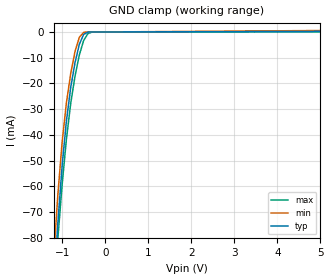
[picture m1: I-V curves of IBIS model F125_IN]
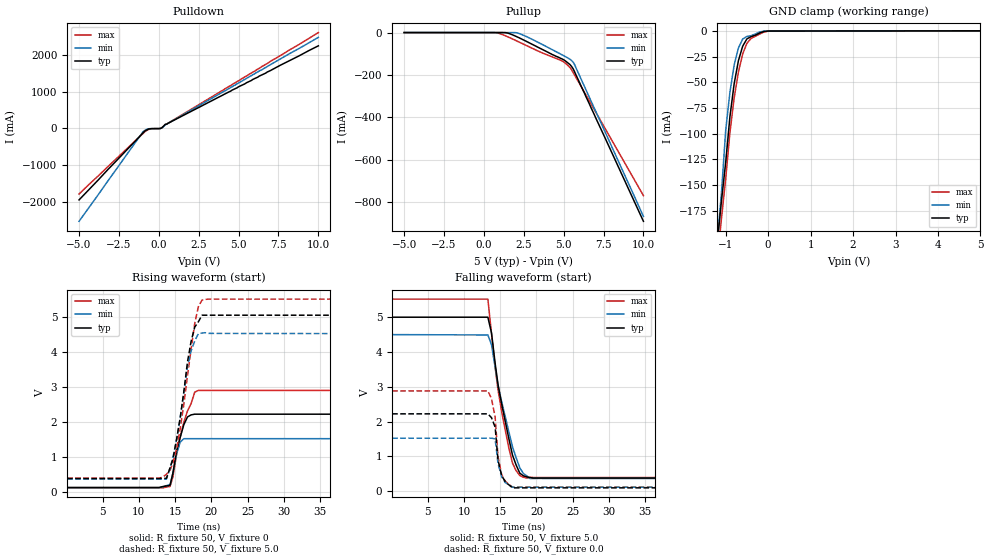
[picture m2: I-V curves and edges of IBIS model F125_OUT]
| TEXAS INSTRUMENTS INCORPORATED
| Standard Linear and Logic Group
| IBIS Model of SN74F125
| QUADRUPLE BUS BUFFER GATE WITH 3-STATE OUTPUTS
| SOIC 14-pin (D),PDIP 14-pin (N), SOP 14-pin (NS) Package.
[IBIS Ver]   3.2
[Comment Char]  |_char
[File Name]   sn74f125.ibs
[File Rev]   3.1
[Date]   Nov. 03, 2004
[Source]   Data created from Lab data at TI-SLL.
[Notes]   The following is an IBIS list for the F125.
   - FILE REV HISTORY
   - 3.1 Re-Release IBIS file on 11/03/04
   - Power clamp data deleted as there is no power-clamp diode.
|   Please contact sllibis@ti.com with questions and
|   comments concerning SLL IBIS models.
[Disclaimer] Property of Texas Instruments Incorporated.  Unauthorized
   reproduction and/or distribution is strictly prohibited.
   This product is protected under copyright law.
   Created 2000, (C) Copyright 2000, Texas Instruments Inc.,
   All Rights Reserved.
   UNLESS THERE IS A SIGNED, WRITTEN AGREEMENT TO THE
   CONTRARY, TEXAS INSTRUMENTS () IS PROVIDING THE IBIS
   MODELS  AND WITHOUT ANY WARRANTY, EXPRESSED OR
   IMPLIED.  TI assumes no liability for:
   1) the accuracy of the IBIS models provided to your
   company;
   2) the proper functioning of these IBIS Models in your
   design or for any resulting applications; or
   3) infringement of patents, copyrights or intellectual
   property rights resulting from your use of these IBIS
   models.
   TI provides IBIS Models as a service to our customers.
   You and your company shall not distribute, sell or give
   these models to anyone else without prior written
   permission from TI.
   TI reserves the right to make changes to our products or
   to discontinue any semiconductor product or service
   without notice, and advises our customers to obtain the
   latest version of relevant information to verify, before
   placing orders, that the information being relied on is
   current.
   Please be aware that your receipt and use of the IBIS
   information provided shall serve as acceptance of these
   terms and conditions.  If you do not accept these terms,
   you should return or destroy the IBIS models and any
   other accompanying information immediately.
|   Component F125_D
[Component]   F125_D
[Manufacturer]  Texas Instruments Incorporated
[Package]
|   Typ.   Min.   Max.
R_pkg   0.031   0.028   0.034
L_pkg   3.109nH   2.462nH   3.889nH
C_pkg   0.473pF   0.363pF   0.628pF
[Pin]   Signal_name   Model_name   R_pin   L_pin   C_pin
1   1OE_NOT   F125_IN   0.033   3.854nH   0.622pF
2   1A   F125_IN   0.032   3.188nH   0.473pF
3   1Y   F125_OUT   0.028   2.462nH   0.377pF
4   2OE_NOT   F125_IN   0.031   2.596nH   0.363pF
5   2A   F125_IN   0.028   2.521nH   0.372pF
6   2Y   F125_OUT   0.034   3.25nH   0.476pF
7   GND   GND   0.034   3.889nH   0.628pF
8   3Y   F125_OUT   0.034   3.889nH   0.628pF
9   3A   F125_IN   0.034   3.25nH   0.476pF
10   3OE_NOT   F125_IN   0.028   2.521nH   0.372pF
11   4Y   F125_OUT   0.031   2.596nH   0.364pF
12   4A   F125_IN   0.028   2.462nH   0.377pF
13   4OE_NOT   F125_IN   0.032   3.188nH   0.473pF
14   VCC   POWER   0.033   3.854nH   0.622pF
|   Component F125_N
[Component]   F125_N
[Manufacturer]  Texas Instruments Incorporated
[Package]
|   Typ.   Min.   Max.
R_pkg   0.045   0.037   0.063
L_pkg   5.407nH   3.922nH   6.942nH
C_pkg   0.389pF   0.205pF   0.604pF
[Pin]  Signal_name   Model_name   R_pin   L_pin   C_pin
1   1OE_NOT   F125_IN   0.063   6.942nH   0.604pF
2   1A   F125_IN   0.037   6.2nH   0.406pF
3   1Y   F125_OUT   0.042   4.389nH   0.322pF
4   2OE_NOT   F125_IN   0.038   3.922nH   0.205pF
5   2A   F125_IN   0.039   4.301nH   0.298pF
6   2Y   F125_OUT   0.038   5.329nH   0.356pF
7   GND   GND   0.053   6.51nH   0.544pF
8   3Y   F125_OUT   0.053   6.437nH   0.539pF
9   3A   F125_IN   0.039   5.352nH   0.347pF
10   3OE_NOT   F125_IN   0.042   4.473nH   0.297pF
11   4Y   F125_OUT   0.044   4.326nH   0.225pF
12   4A   F125_IN   0.042   4.295nH   0.28pF
13   4OE_NOT   F125_IN   0.042   6.318nH   0.418pF
14   VCC   POWER   0.061   6.9nH   0.603pF
|   Component F125_NS
[Component]   F125_NS
[Manufacturer]  Texas Instruments, Inc.
[Package]
|   typ   min   max
R_pkg   4.500e-02   3.900e-02   5.400e-02
L_pkg   3.796e-09   2.561e-09   4.952e-09
C_pkg   5.280e-13   2.880e-13   7.100e-13
[Pin]   signal_name   model_name   R_pin   L_pin   C_pin
1   1OE_NOT   F125_IN   4.700e-02   4.867e-09   7.060e-13
2   1A   F125_IN   5.100e-02   4.083e-09   5.920e-13
3   1Y   F125_OUT   4.100e-02   2.915e-09   3.760e-13
4   2OE_NOT   F125_IN   3.900e-02   2.561e-09   2.880e-13
5   2A   F125_IN   4.100e-02   3.101e-09   4.300e-13
6   2Y   F125_OUT   4.700e-02   4.047e-09   5.890e-13
7   GND   GND   5.100e-02   4.909e-09   7.000e-13
8   3Y   F125_OUT   4.500e-02   4.784e-09   6.940e-13
9   3A   F125_IN   5.400e-02   4.176e-09   5.970e-13
10   3OE_NOT   F125_IN   3.900e-02   3.287e-09   4.490e-13
11   4Y   F125_OUT   3.900e-02   2.586e-09   2.940e-13
12   4A   F125_IN   4.000e-02   2.802e-09   3.710e-13
13   4OE_NOT   F125_IN   4.900e-02   4.080e-09   5.930e-13
14   VCC   POWER   5.200e-02   4.952e-09   7.100e-13
| Models and submodels in the file (2): F125_IN (Input), F125_OUT (3-state)
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|   Model F125_IN
[Model]   F125_IN
Model_type  Input
Polarity   Inverting
Vinl = 0.8
Vinh = 2.0
| variable   typ   min   max
C_comp   1.24pf   0.94pf   1.54pf
[Temperature Range]   25   0   70
[Voltage Range]   5.0   4.5   5.5
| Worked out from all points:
|   GND clamp passes 1 mA (typ) near -0.50 V on its own axis
[GND Clamp]
|   Voltage   I(typ)   I(min)   I(max)
-5V       -1.74A     -1.55A     -1.51A
-1.2V     -101mA     -88.7mA    -104mA
-1.1V     -74.4mA    -63.5mA    -80.4mA
-1V       -52mA      -42.8mA    -59.4mA
-900mV    -34.5mA    -27.5mA    -41.6mA
-800mV    -21.5mA    -16.1mA    -27.7mA
-700mV    -11.9mA    -7.52mA    -17.1mA
-600mV    -4.79mA    -2.08mA    -8.9mA
-500mV    -950uA     -140uA     -3.31mA
-400mV    -55.2uA    -3.23uA    -617uA
-300mV    -1.95uA    -61.9nA    -49uA
5V        230uA      555uA      4.72uA
|   Model F125_OUT
[Model]   F125_OUT
Model_type  3-state
Polarity   Non-Inverting
Enable   Active-High
Vmeas = 2.5v
Cref = 15pf
| variable   typ   min   max
C_comp   6.5pf   4.87pf   8.13pf
[Temperature Range]   25   0   70
[Voltage Range]   5.0   4.5   5.5
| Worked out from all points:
|   slope of the pulldown table from 0 to 0.75 V, typ, clamps not added: 4.12 ohm
|   GND clamp passes 1 mA (typ) near -0.14 V on its own axis
|   rising waveform, R_fixture 50, V_fixture 0: 20-80 % time 1.33ns typ, 901ps min, 1.89ns max; typ from 0.125 V to 2.22 V
|   falling waveform, R_fixture 50, V_fixture 5.0: 20-80 % time 2.34ns typ, 2.62ns min, 2.2ns max; typ from 5 V to 0.373 V
|   rising waveform, R_fixture 50, V_fixture 5.0: 20-80 % time 2.01ns typ, 1.92ns min, 2.12ns max; typ from 0.383 V to 5.05 V
|   falling waveform, R_fixture 50, V_fixture 0.0: 20-80 % time 802ps typ, 804ps min, 899ps max; typ from 2.22 V to 0.092 V
[Pulldown]
|   Voltage   I(typ)   I(min)   I(max)
-5V       -1.94A     -2.52A     -1.78A
-1V       -127mA     -96.6mA    -143mA
-900mV    -82mA      -59.8mA    -98.3mA
-600mV    -14.2mA    -7.87mA    -22.4mA
100mV     -1.69mA    -3.1mA     291uA
200mV     19.5mA     12.8mA     23.8mA
400mV     108mA      101mA      106mA
500mV     117mA      114mA      116mA
10V       2.24A      2.47A      2.6A
[Pullup]
|   Voltage   I(typ)   I(min)   I(max)
-5V       59.3nA     2nA        697nA
700mV     -327nA     1.56nA     -184uA
1.4V      -873uA     -817nA     -16.9mA
2V        -17.4mA    -408uA     -37.3mA
2.5V      -35.3mA    -13.3mA    -55.1mA
3.7V      -80.9mA    -57.7mA    -97mA
4.8V      -121mA     -101mA     -130mA
5V        -128mA     -109mA     -138mA
5.4V      -151mA     -126mA     -165mA
5.6V      -171mA     -140mA     -189mA
5.7V      -187mA     -153mA     -202mA
10V       -889mA     -866mA     -768mA
[GND Clamp]
|   Voltage   I(typ)   I(min)   I(max)
-5V       -1.73A     -2.07A     -1.79A
-1.2V     -207mA     -206mA     -225mA
-1.1V     -166mA     -158mA     -183mA
-1V       -128mA     -96.9mA    -144mA
-900mV    -83.5mA    -59.6mA    -98.9mA
-800mV    -51.3mA    -33.1mA    -65.1mA
-700mV    -28.9mA    -16.6mA    -40mA
-600mV    -14.8mA    -7.84mA    -22.4mA
-500mV    -7.66mA    -5.27mA    -12mA
-400mV    -5.47mA    -4.55mA    -7.11mA
0V        -32.9uA    -3.23uA    -149uA
5V        201uA      174uA      8.82uA
[Ramp]
| variable   typ   min   max
dV/dt_r   1.30E+00/1.18E-10   1.06E+00/1.16E-09   1.44E+00/1.19E-10
dV/dt_f   2.89E+00/1.74E-10   2.60E+00/2.08E-09   2.97E+00/1.43E-10
R_load = 50
[Rising Waveform]
R_fixture = 50
V_fixture = 0
|   Time   V(typ)   V(min)   V(max)
97.7ps    125mV      116mV      114mV
12.8ns    125mV      116mV      114mV
14.3ns    186mV      201mV      154mV
14.7ns    540mV      537mV      430mV
15.2ns    1.17V      1.08V      1.08V
15.7ns    1.56V      1.42V      1.56V
16.7ns    2.14V      1.52V      2.31V
17.7ns    2.22V      1.52V      2.85V
18.2ns    2.22V      1.52V      2.9V
49.8ns    2.22V      1.52V      2.9V
[Falling Waveform]
R_fixture = 50
V_fixture = 5.0
V_fixture_min = 4.5
V_fixture_max = 5.5
|   Time   V(typ)   V(min)   V(max)
97.7ps    5V         4.5V       5.52V
13.3ns    5V         4.49V      5.52V
13.8ns    4.55V      4.21V      4.53V
14.7ns    3.06V      3.04V      2.91V
15.7ns    2V         2.14V      1.75V
16.7ns    1.03V      1.27V      802mV
17.7ns    514mV      667mV      448mV
18.2ns    439mV      504mV      396mV
19.1ns    389mV      360mV      393mV
49.8ns    373mV      361mV      390mV
[Rising Waveform]
R_fixture = 50
V_fixture = 5.0
V_fixture_min = 4.5
V_fixture_max = 5.5
|   Time   V(typ)   V(min)   V(max)
97.7ps    383mV      360mV      390mV
13.8ns    386mV      363mV      500mV
14.3ns    690mV      676mV      619mV
14.7ns    938mV      977mV      830mV
15.7ns    2.12V      2.11V      1.81V
16.7ns    3.71V      3.57V      3.32V
17.2ns    4.3V       4.03V      4.07V
18.2ns    4.86V      4.52V      5.29V
18.7ns    5.05V      4.54V      5.48V
49.8ns    5.05V      4.52V      5.51V
[Falling Waveform]
R_fixture = 50
V_fixture = 0.0
|   Time   V(typ)   V(min)   V(max)
97.7ps    2.22V      1.52V      2.88V
13.3ns    2.22V      1.52V      2.88V
13.8ns    2.11V      1.52V      2.66V
14.3ns    1.84V      1.5V       2.13V
14.7ns    890mV      789mV      993mV
15.2ns    448mV      411mV      469mV
15.7ns    265mV      242mV      283mV
16.7ns    91.6mV     112mV      110mV
49.8ns    91.6mV     112mV      110mV
